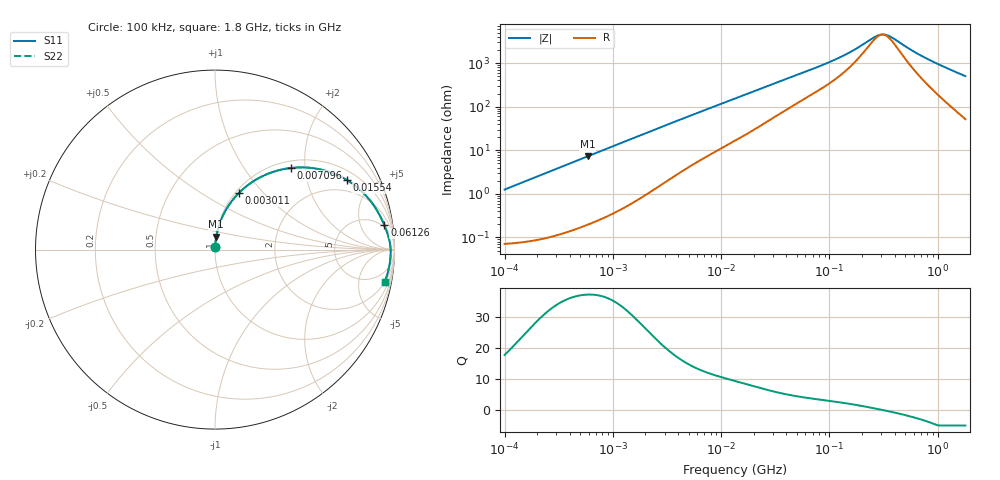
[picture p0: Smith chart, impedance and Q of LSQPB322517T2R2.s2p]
! LSQPB322517T2R2  S-PARAMETER MODEL  ( General Type )
! Model Generated by TAIYO YUDEN Corporation (http://www.ty-top.com)
! Version 2.0
! TAIYO YUDEN Control No. 100810NC14SB-FKC
! Copyright(c) 2008 TAIYO YUDEN CO.,LTD. All Rights Reserved.
! Product Description (link to TY-COMPAS)
! https://ds.yuden.co.jp/TYCOMPAS/or/detail?pn=LSQPB322517T2R2M&u=M
! Products Name : Inductors
! Characteristics :
!  Inductance : 2.2 uH , SRF(min) : 150 MHz , DC Resistance(max) : 0.078 Ohm
!  Rated Current : Saturation :1850 mA , Temp Rise : 1600 mA (40 degC)
!  Case Size : 3.2 x 2.5 / 0.126 x 0.098 [mm/inch] , Thickness : 1.7 / 0.068 [mm/inch]
!  (Conditions: Temperature = 25 degC , DC Bias Current/Voltage = 0A / 0V)
! External Node Assignments :
!  1  o---GGG---o  2
! GND o---------o GND
! Frequency Range : 0.1MHz  -  1800MHz  [ 402 STEP ]
# MHz S RI R 50
! Freq[MHz].  S11 Real  S11 Imag  S21 Real  S21 Imag  S12 Real  S12 Imag  S22 Real  S22 Imag
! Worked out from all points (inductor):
!   401 points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, 100 kHz to 1.8 GHz, reference 50 ohm
!   read as one part in series: L = 2 uH near 105 kHz
!   highest Q = 37.1 at 583.4 kHz (marker M1), where L = 1.98 uH
!   self-resonance near 307.4 MHz
!   S11 on the Smith chart (normalised r, x): 100 kHz: 1.00, +0.03; 3.011 MHz: 1.04, +0.73; 7.096 MHz: 1.14, +1.68; 15.54 MHz: 1.41, +3.53; 61.26 MHz: 4, +13; 1.8 GHz: 2, -10
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0.1  0.000867 0.0125  0.9991 -0.0125  0.9991 -0.0125  0.000867 0.0125
0.516129  0.00583 0.0638  0.9942 -0.0638  0.9942 -0.0638  0.00583 0.0638
0.583377  0.00716 0.0719  0.9928 -0.0719  0.9928 -0.0719  0.00716 0.0719
1.443982  0.036 0.1707  0.964 -0.1707  0.964 -0.1707  0.036 0.1707
2.66389  0.1068 0.2868  0.8932 -0.2868  0.8932 -0.2868  0.1068 0.2868
3.010975  0.131 0.3135  0.869 -0.3135  0.869 -0.3135  0.131 0.3135
4.455722  0.2386 0.3956  0.7614 -0.3956  0.7614 -0.3956  0.2386 0.3956
7.096489  0.4208 0.4546  0.5792 -0.4546  0.5792 -0.4546  0.4208 0.4546
9.75753  0.5596 0.4518  0.4404 -0.4518  0.4404 -0.4518  0.5596 0.4518
13.41641  0.6866 0.4132  0.3134 -0.4132  0.3134 -0.4132  0.6866 0.4132
15.54051  0.7366 0.3866  0.2634 -0.3866  0.2634 -0.3866  0.7366 0.3866
27.97575  0.8722 0.2633  0.1278 -0.2633  0.1278 -0.2633  0.8722 0.2633
61.26374  0.9437 0.1357  0.0563 -0.1357  0.0563 -0.1357  0.9437 0.1357
69.24595  0.9496 0.1212  0.0504 -0.1212  0.0504 -0.1212  0.9496 0.1212
140.897  0.971 0.0544  0.029 -0.0544  0.029 -0.0544  0.971 0.0544
272.9811  0.978 0.00783  0.022 -0.00783  0.022 -0.00783  0.978 0.00783
308.5485  0.9785 -0.000238  0.0215 0.000238  0.0215 0.000238  0.9785 -0.000238
357.3983  0.9788 -0.00999  0.0212 0.00999  0.0212 0.00999  0.9788 -0.00999
569.2172  0.9776 -0.0435  0.0224 0.0435  0.0224 0.0435  0.9776 -0.0435
745.2431  0.9752 -0.0667  0.0248 0.0667  0.0248 0.0667  0.9752 -0.0667
1158.204  0.9661 -0.1152  0.0339 0.1152  0.0339 0.1152  0.9661 -0.1152
1800  0.9445 -0.1829  0.0555 0.1829  0.0555 0.1829  0.9445 -0.1829
